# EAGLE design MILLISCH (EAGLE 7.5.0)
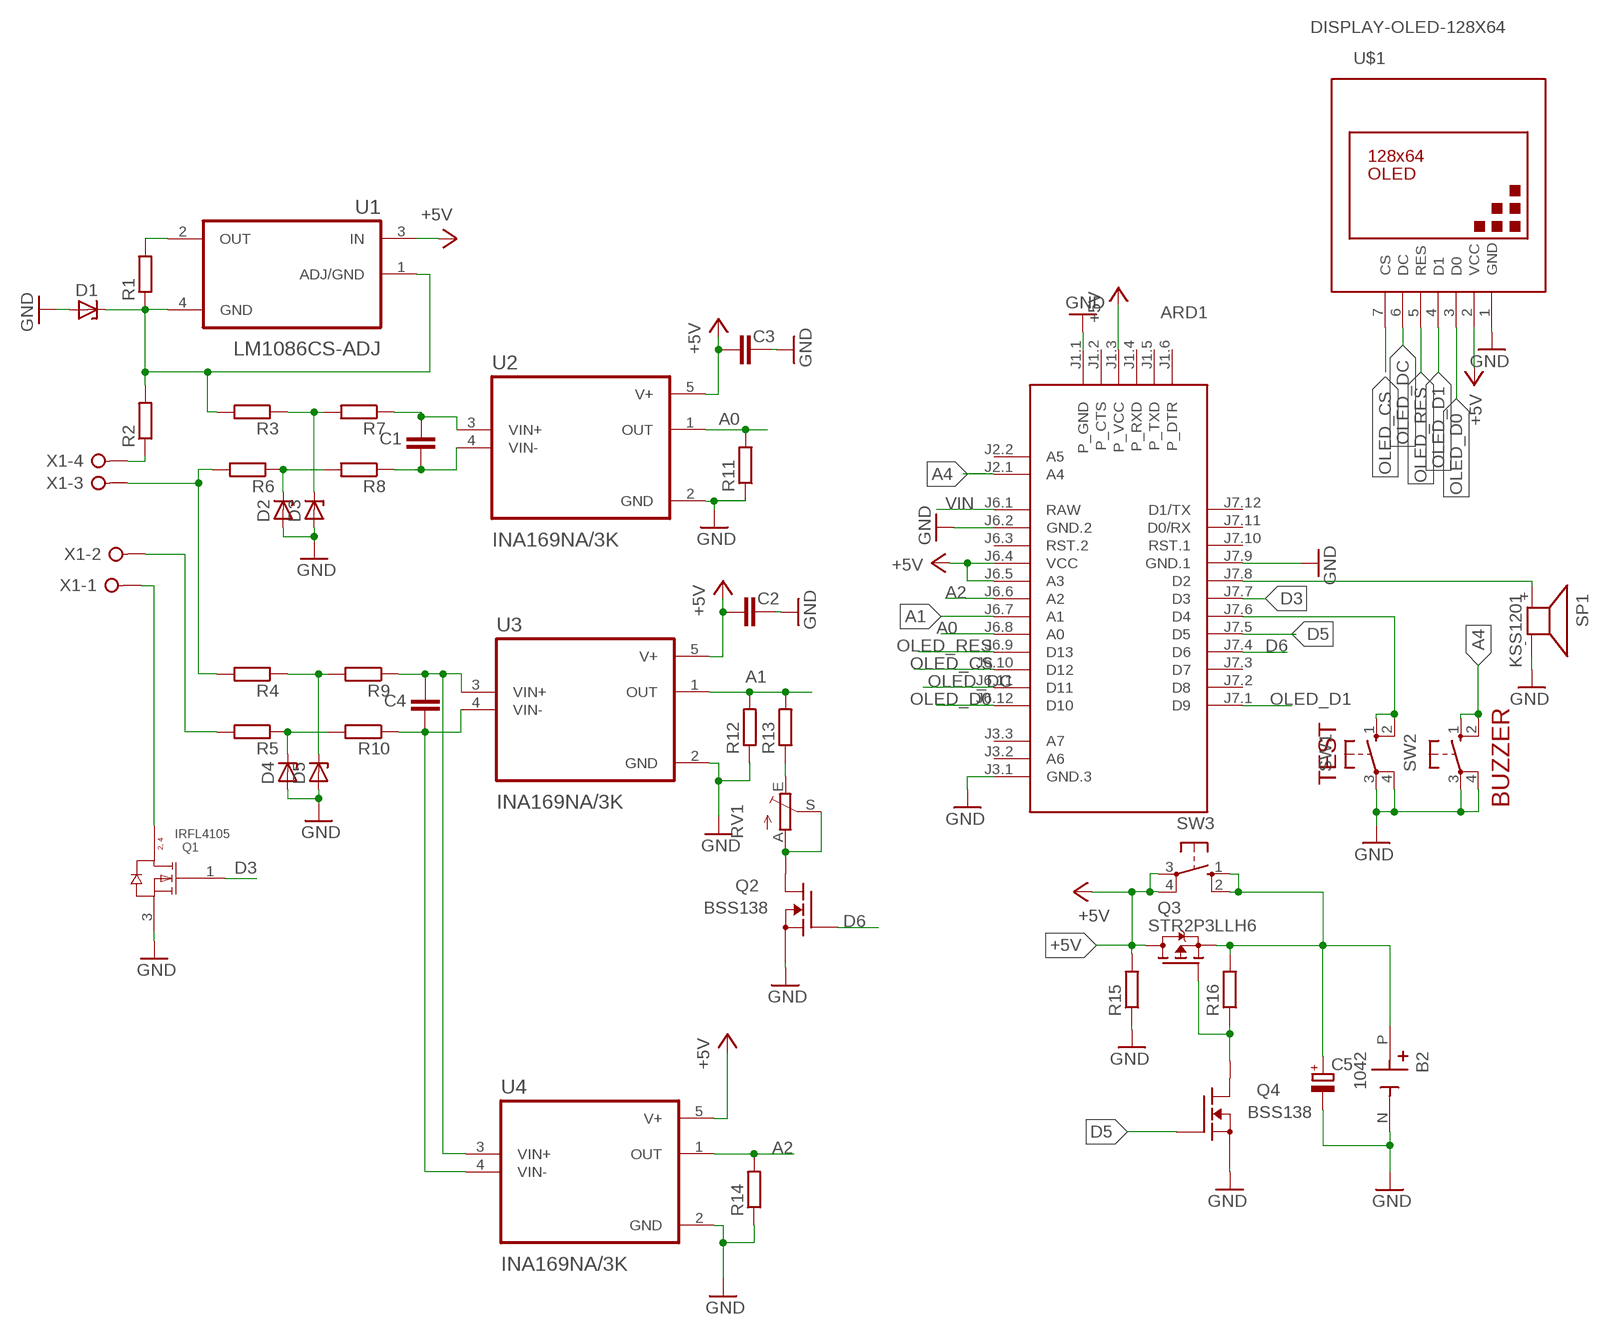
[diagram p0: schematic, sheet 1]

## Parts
ARD1  ARDUINO-PRO-MINI-3.3V  [ARDUINO-PRO-MINI]
B2  1042  [BAT_1042]
C1  C-EUC0805  [C0805]
C2  C-EUC0805  [C0805]
C3  C-EUC0805  [C0805]
C4  C-EUC0805  [C0805]
C5  CPOL-EUSMCD  [SMC_D]
D1  ZENER-DIODESMB  [SMB]
D2  ZENER-DIODESMB  [SMB]
D3  ZENER-DIODESMB  [SMB]
D4  ZENER-DIODESMB  [SMB]
D5  ZENER-DIODESMB  [SMB]
Q1  IRFL4105  NTF3055L108T1GNTF3055L108T1G_ONSC-SOT-223-4-318E-04_V  [ONSC-SOT-223-4-318E-04_V]
Q2  BSS138  [SOT23]
Q3  STR2P3LLH6  [SOT23]
Q4  BSS138  [SOT23]
R1  R-EU_R2512  [R2512]
R2  R-EU_R2512  [R2512]
R3  R-EU_R2512  [R2512]
R4  R-EU_R2512  [R2512]
R5  R-EU_R2512  [R2512]
R6  R-EU_R2512  [R2512]
R7  R-EU_R0805  [R0805]
R8  R-EU_R0805  [R0805]
R9  R-EU_R0805  [R0805]
R10  R-EU_R0805  [R0805]
R11  R-EU_R0805  [R0805]
R12  R-EU_R0805  [R0805]
R13  R-EU_R0805  [R0805]
R14  R-EU_R0805  [R0805]
R15  R-EU_R0805  [R0805]
R16  R-EU_R0805  [R0805]
RV1  TRIM_EU-B64W  [B64W]
SP1  KSS1201  [KSS1201]
SW1  10-XX  [B3F-10XX]
SW2  10-XX  [B3F-10XX]
SW3  10-XX  [B3F-10XX]
U1  LM1086CS-ADJ  [TO254P1524X483-4N]
U2  INA169NA/3K  [SOT95P280X145-5N]
U3  INA169NA/3K  [SOT95P280X145-5N]
U4  INA169NA/3K  [SOT95P280X145-5N]
U$1  DISPLAY-OLED-128X64  [DISPLAY-OLED-128X64]
X1  W237-04P  [W237-4P]

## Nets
+5V: ARD1.J1.3(P_VCC) ARD1.J6.4(VCC) ARD1.J6.5(A3) C2.1 C3.1 Q3.1(D) R15.2 SW3.3(P) SW3.4(P1) U1.3(IN) U2.5(V+) U3.5(V+) U4.5(V+) U$1.2(VCC)
A0: ARD1.J6.8(A0) R11.2 U2.1(OUT)
A1: ARD1.J6.7(A1) R12.2 R13.2 U3.1(OUT)
A2: ARD1.J6.6(A2) R14.2 U4.1(OUT)
A4: ARD1.J2.1(A4) SW2.1(S) SW2.2(S1)
D3: ARD1.J7.7(D3) Q1.1(G)
D5: ARD1.J7.5(D5) Q4.3(G)
D6: ARD1.J7.4(D6) Q2.3(G)
GND: ARD1.J1.1(P_GND) ARD1.J3.1(GND.3) ARD1.J6.2(GND.2) ARD1.J7.9(GND.1) B2.N(NEG) C2.2 C3.2 C5.- D1.A D2.A D3.A D4.A D5.A Q1.3(S) Q2.1(S) Q4.1(S) R11.1 R12.1 R14.1 R15.1 SP1.- SW1.3(P) SW1.4(P1) SW2.3(P) SW2.4(P1) U2.2(GND) U3.2(GND) U4.2(GND) U$1.1(GND)
N$1: C1.1 R7.1 U2.3(VIN+)
N$2: C1.2 R8.1 U2.4(VIN-)
N$3: R1.2 U1.2(OUT)
N$4: D1.C R1.1 R2.2 R3.2 U1.1(ADJ/GND) U1.4(GND)
N$5: R2.1 X1.4
N$6: R4.2 R6.2 X1.3
N$7: D3.C R3.1 R7.2
N$8: Q1.4(D) X1.1
N$9: D2.C R6.1 R8.2
N$10: C4.2 R10.1 U3.4(VIN-) U4.4(VIN-)
N$11: D5.C R4.1 R9.2
N$12: D4.C R5.1 R10.2
N$13: R5.2 X1.2
N$14: C4.1 R9.1 U3.3(VIN+) U4.3(VIN+)
N$15: Q2.2(D) RV1.A RV1.S
N$16: R13.1 RV1.E
N$17: ARD1.J7.8(D2) SP1.+
N$18: ARD1.J7.6(D4) SW1.1(S) SW1.2(S1)
N$19: Q3.2(G) Q4.2(D) R16.1
N$20: B2.P(POS) C5.+ Q3.3(S) R16.2 SW3.1(S) SW3.2(S1)
OLED_CS: ARD1.J6.10(D12) U$1.7(CS)
OLED_D0: ARD1.J6.12(D10) U$1.3(D0)
OLED_D1: ARD1.J7.1(D9) U$1.4(D1)
OLED_DC: ARD1.J6.11(D11) U$1.6(DC)
OLED_RES: ARD1.J6.9(D13) U$1.5(RES)
VIN: ARD1.J6.1(RAW)
Unconnected: ARD1.J1.2(P_CTS) ARD1.J1.4(P_RXD) ARD1.J1.5(P_TXD) ARD1.J1.6(P_DTR) ARD1.J2.2(A5) ARD1.J3.2(A6) ARD1.J3.3(A7) ARD1.J6.3(RST.2) ARD1.J7.2(D8) ARD1.J7.3(D7) ARD1.J7.10(RST.1) ARD1.J7.11(D0/RX) ARD1.J7.12(D1/TX) Q1.2(D)

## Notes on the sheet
- TEST
- BUZZER

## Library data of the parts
ARD1 = diy-modules:ARDUINO-PRO-MINI-*: Arduino Pro Mini and compatible devices More details available here: https://www.arduino.cc/en/Main/ArduinoBoardProMini Click here to find device on ebay.com
B2 = 18650-HOLDER:1042: Check availability; AVAILABILITY: In Stock; CHECK_PRICES: https://www.snapeda.com/parts/1042/Keystone/view-part/?ref=eda; DESCRIPTION: SMT Holder for 18650 Battery; MF: Keystone Electronics Corp.; MP: 1042; PACKAGE: NON STANDARD-5 Keystone; PRICE: None; SNAPEDA_LINK: https://www.snapeda.com/parts/1042/Keystone/view-part/?ref=snap
C1-C4 = rcl:C-EU: CAPACITOR, European symbol
C5 = rcl:CPOL-EU: POLARIZED CAPACITOR, European symbol
D1-D5 = diode:ZENER-DIODE: Z-Diode
Q1 = NTF3055L108T1G:NTF3055L108T1G: Power MOSFET, 3 A, 60 V, Logic Level, N-Channel, 4-Pin SOT-223, Pb-Free, Tape and Reel Check availability; AVAILABILITY: In Stock; CHECK_PRICES: https://www.snapeda.com/parts/NTF3055L108T1G/Onsemi/view-part/?ref=eda; DESCRIPTION: N-Channel 60 V 3A (Ta) 1.3W (Ta) Surface Mount SOT-223 (TO-261); MF: ON Semiconductor; MP: NTF3055L108T1G; PACKAGE: SOT-223-4 ON Semiconductor; PRICE: None; SNAPEDA_LINK: https://www.snapeda.com/parts/NTF3055L108T1G/Onsemi/view-part/?ref=snap
Q2 Q4 = transistor-fet:BSS138
Q3 = transistor-fet:STR2P3LLH6
R1-R16 = rcl:R-EU_: RESISTOR, European symbol
RV1 = pot:TRIM_EU-: POTENTIOMETER
SP1 = buzzer:KSS1201: SPEAKER; OC_FARNELL: unknown; OC_NEWARK: unknown
SW1-SW3 = switch-omron:10-XX: OMRON SWITCH; MPN: B3F-1000; OC_FARNELL: 176432; OC_NEWARK: 36M3542
U1 = LM1086CS-ADJ:LM1086CS-ADJ: Check availability; AVAILABILITY: In Stock; CHECK_PRICES: https://www.snapeda.com/parts/LM1086CS-ADJ/NOPB/Texas+Instruments/view-part/?ref=eda; DESCRIPTION: 1.5-A, 29-V, linear voltage regulator; MF: Texas Instruments; MP: LM1086CS-ADJ/NOPB; PACKAGE: TO263-3 Texas Instruments; PRICE: None; SNAPEDA_LINK: https://www.snapeda.com/parts/LM1086CS-ADJ/NOPB/Texas+Instruments/view-part/?ref=snap
U2-U4 = INA169NA_3K:INA169NA/3K: Check availability; AVAILABILITY: In Stock; CHECK_PRICES: https://www.snapeda.com/parts/INA169NA/3K/Texas+Instruments/view-part/?ref=eda; DESCRIPTION: 2.7 to 60V, 440kHz Variable gain current sense amplifier; MF: Texas Instruments; MP: INA169NA/3K; PACKAGE: SOT-23-5 Texas Instruments; PRICE: None; PURCHASE-URL: https://pricing.snapeda.com/search?q=INA169NA/3K&ref=eda; SNAPEDA_LINK: https://www.snapeda.com/parts/INA169NA/3K/Texas+Instruments/view-part/?ref=snap
U$1 = diy-modules:DISPLAY-OLED-128X64: 128x64 Dot Matrix OLED Module based on SSD1306 chip Variant with SPI interface More details available here: http://www.instructables.com/id/How-to-use-OLED-display-arduino-module/ SSD1306 datasheet: https://cdn-shop.adafruit.com/datasheets/SSD1306.pdf Click here to find device on ebay.com Note: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
X1 = con-wago-508:W237-04P: WAGO SREW CLAMP; OC_FARNELL: unknown; OC_NEWARK: unknown

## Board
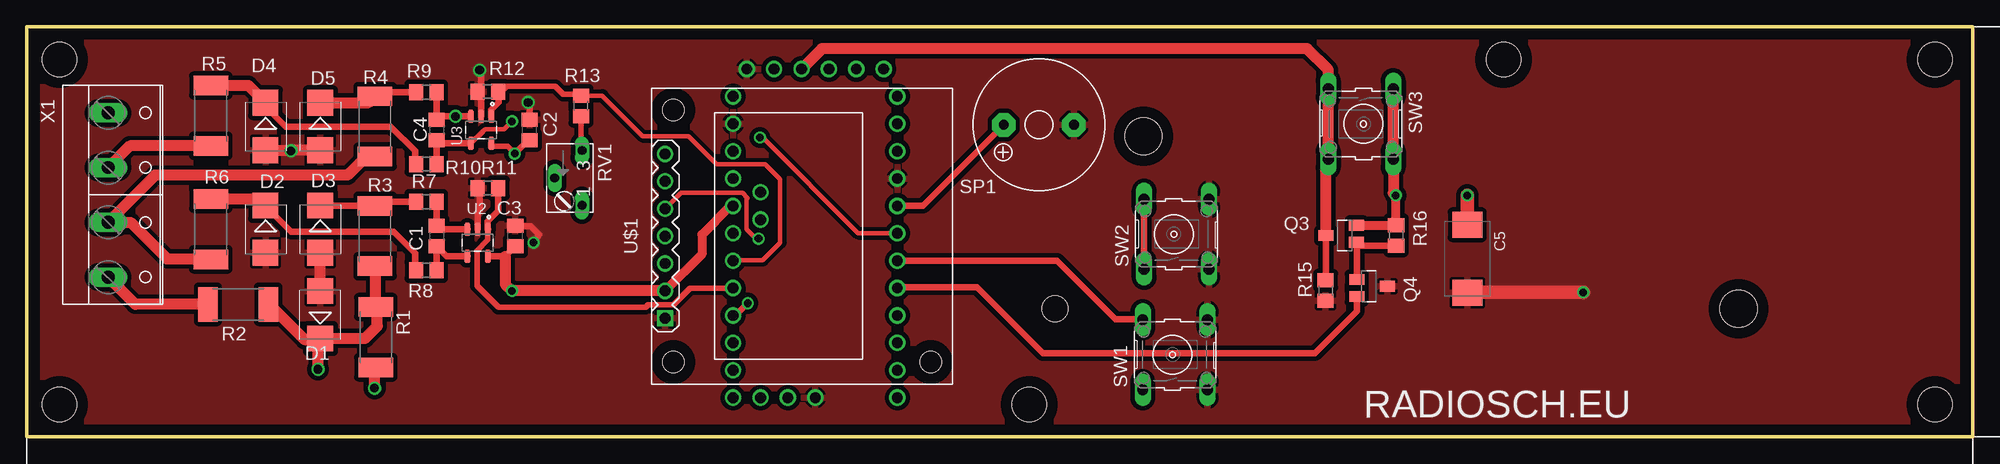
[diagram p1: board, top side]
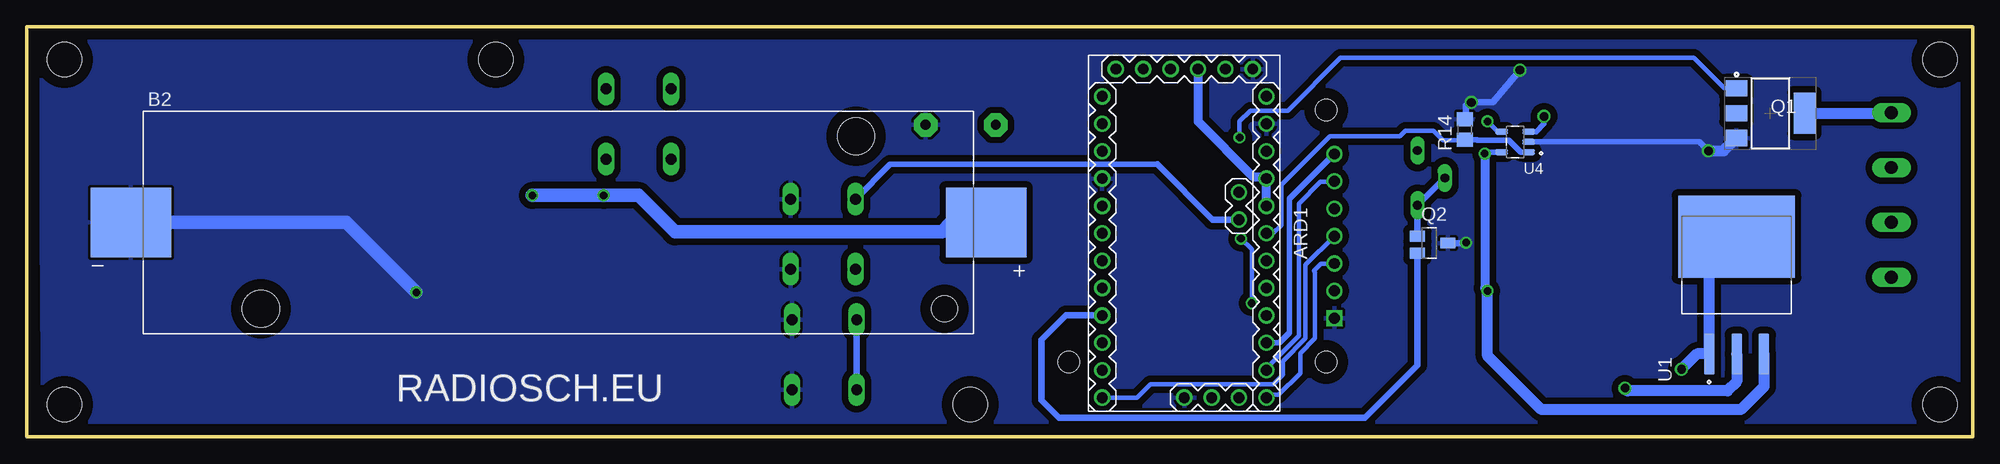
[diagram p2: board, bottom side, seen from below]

Size 180.5 x 38 mm. Coordinates in mm from the lower left corner, seen from the top.
Outline: 0,0 180.5,0 180.5,38 0,38 0,0
Copper layers (1*16): Top 0.035mm / dielectric 1.5mm / Bottom 0.035mm
Design rules "default": minimum track width 10mil, minimum drill 24mil, track to track 8mil, track to pad 8mil, pad to pad 8mil, via to via 8mil, smd to smd 8mil, copper to edge 40mil, drill to drill 8mil, minimum pad ring 10mil, minimum via ring 8mil, stop-mask expansion 4mil, vias tented up to drill 0mil, thermal gap 10mil
Holes 3.2 mm at 3,35 3,3 93,3 177,3 177,35 137,35

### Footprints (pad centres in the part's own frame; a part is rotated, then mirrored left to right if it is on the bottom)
ARDUINO-PRO-MINI = drill 1: J1.1 -15.24,6.35; J1.2 -15.24,3.81; J1.3 -15.24,1.27; J1.4 -15.24,-1.27; J1.5 -15.24,-3.81; J1.6 -15.24,-6.35; J2.1 -1.27,5.08; J2.2 -3.81,5.08; J3.1 15.24,0; J3.2 15.24,2.54; J3.3 15.24,5.08; J6.1 -12.7,7.62; J6.2 -10.16,7.62; J6.3 -7.62,7.62; J6.4 -5.08,7.62; J6.5 -2.54,7.62; J6.6 0,7.62; J6.7 2.54,7.62; J6.8 5.08,7.62; J6.9 7.62,7.62; J6.10 10.16,7.62; J6.11 12.7,7.62; J6.12 15.24,7.62; J7.1 15.24,-7.62; J7.2 12.7,-7.62; J7.3 10.16,-7.62; J7.4 7.62,-7.62; J7.5 5.08,-7.62; J7.6 2.54,-7.62; J7.7 0,-7.62; J7.8 -2.54,-7.62; J7.9 -5.08,-7.62; J7.10 -7.62,-7.62; J7.11 -10.16,-7.62; J7.12 -12.7,-7.62
BAT_1042 = smd 7.46 x 6.47: N -39.67,0; P 39.67,0 | hole 3.45: 27.6,8; -27.6,-8 | hole 2.39: 35.82,-8
C0805 = smd 1.3 x 1.5: 1 -0.95,0; 2 0.95,0
SMC_D = smd 2.4 x 2.8: + -3.15,0; - 3.15,0
SMB = smd 2.4 x 2.4: A 2.2,0; C -2.2,0
ONSC-SOT-223-4-318E-04_V = smd 2 x 1.5: 1 -3.15,2.3; 2 -3.15,0; 3 -3.15,-2.3 | smd 2 x 3.8: 4 3.15,0
SOT23 = smd 1 x 1.4: 1 0,1.735; 2 -0.632,-1.1; 3 0.95,-1.1
R2512 = smd 1.8 x 3.2: 1 -2.8,0; 2 2.8,0
R0805 = smd 1.3 x 1.5: 1 -0.95,0; 2 0.95,0
B64W = drill 0.813 long: A 2.54,0; E -2.54,0; S 0,-2.54
KSS1201 = drill 0.914 pad 2.159 octagon: + 3.251,0; - -3.251,0
B3F-10XX = drill 1.016 long: 1 -3.251,2.761; 2 3.251,2.761; 3 -3.251,-3.261; 4 3.251,-3.261
TO254P1524X483-4N = smd 3.79 x 0.99: 1 -6.4,2.54; 2 -6.4,0; 3 -6.4,-2.54 | smd 7.62 x 10.84: 4 4.48,0
SOT95P280X145-5N = smd 1.21 x 0.59: 1 -1.255,0.95; 2 -1.255,0; 3 -1.255,-0.95; 4 1.255,-0.95; 5 1.255,0.95
DISPLAY-OLED-128X64 = drill 1 square: 1 -7.62,12.7 | drill 1: 2 -5.08,12.7; 3 -2.54,12.7; 4 0,12.7; 5 2.54,12.7; 6 5.08,12.7; 7 7.62,12.7 | hole 2: -11.684,11.938; 11.684,11.938; -11.684,-11.938
W237-4P = drill 1.194 long: 1 -7.62,-0.635; 2 -2.54,-0.635; 3 2.54,-0.635; 4 7.62,-0.635

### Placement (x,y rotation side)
ARD1  73.13,18.86 270 bottom
B2  131.19,19.87 0 bottom
C1  38.01,18.61 270 top
C2  46.62,28.45 90 top
C3  45.31,18.61 90 top
C4  38.01,28.45 270 top
C5  133.62,16.5 270 top
D1  27.21,11.31 90 top
D2  22.13,19.25 270 top
D3  27.21,19.25 270 top
D4  22.13,28.77 270 top
D5  27.21,28.77 270 top
Q1  18.75,30 0 bottom
Q2  50.41,17.95 270 bottom
Q3  122.25,18.66 90 top
Q4  124.48,13.95 270 top
R1  32.37,9.22 270 top
R2  19.59,12.26 0 top
R3  32.29,18.61 270 top
R4  32.29,28.77 270 top
R5  17.05,29.77 270 top
R6  17.05,19.25 270 top
R7  37.05,21.79 180 top
R8  37.05,15.44 180 top
R9  37.05,31.95 180 top
R10  37.05,25.28 180 top
R11  42.77,23.05 0 top
R12  42.75,32 0 top
R13  51.4,30.68 90 top
R14  47.11,28.47 270 bottom
R15  120.47,13.54 90 top
R16  127.02,18.67 90 top
RV1  51.5,24 270 top
SP1  93.88,28.91 180 top
SW1  106.28,7.61 90 top
SW2  106.4,18.79 90 top
SW3  124,29 270 top
U1  21.89,14.07 90 bottom
U2  41.81,17.98 270 top
U3  42.13,28.45 270 top
U4  42.44,27.34 180 bottom
U$1  71.91,18.6 90 top
X1  8.16,22.42 270 top

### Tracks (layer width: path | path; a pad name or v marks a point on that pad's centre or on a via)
+5V  (via drill 0.7)
  Top 0.5: 43.08,26.92 44.58,26.92 v45.25,26.25 46.5,27.5 C2.1
  Top 0.61: U2.5 44.37,16.72 C3.1 | U3.5 43.08,26.92 | Q3.1 120.52,14.54 R15.2
  Top 0.813: ARD1.J6.5 65.28,21.4 62.62,18.75 62.62,16.94 U$1.2
  Top 1.016: 44.37,16.72 44.37,14.15 v45,13.52 U$1.2 | ARD1.J1.3 73.76,36 118.75,36 120.74,34.01 SW3.3 SW3.4 120.52,25.53 Q3.1
  Bottom 0.5: U4.5 45.11,26.39 v45.25,26.25
  Bottom 0.813: v45.25,26.25 45.25,13.77 v45,13.52 | ARD1.J6.5 ARD1.J6.4 65.69,24.12 66.75,24.12 71.86,29.23 ARD1.J1.3
  Bottom 1.016: U1.3 19.35,4.65 21.5,2.5 40,2.5 45,7.5 v45,13.52
A0
  Top 0.5: ARD1.J6.8 61.53,13.78 60,12.25 57.62,12.25 57.38,12 43.75,12 41.75,14 41.75,17.25 42.75,18.25 42.75,19.21 U2.1
  Top 0.61: R11.2 43.72,20.97 42.75,20 42.75,19.25 U2.1
A1
  Top 0.406: R13.2 53.37,31.63 57.12,27.88 61.38,27.88 64,25.25 68.5,25.25 69.88,23.88 69.88,18 68.25,16.38 65.56,16.38 ARD1.J6.7
  Top 0.5: 43.75,31.95 43.95,31.95 44.5,32.5 49,32.5 49.75,31.75 51.28,31.75 R13.2
  Top 0.61: U3.1 43.08,30.33 43.75,31 43.75,31.95 R12.2
A2
  Bottom 0.406: ARD1.J6.6 64.89,18.86 64.12,19.62 64.12,23.38 59.62,27.88 53.12,27.88 52.62,28.38 50,28.38 49.12,27.5 47.13,27.5 R14.2
  Bottom 0.5: R14.2 45.98,27.52 45.96,27.5 43,27.5 41.89,26.39 U4.1
A4
  Top 0.61: SW2.2 SW2.1
  Bottom 0.5: 75.62,25.25 100.43,25.25 SW2.2
  Bottom 0.61: ARD1.J2.1 70.5,20.13 75.62,25.25
D3  (via drill 0.7)
  Top 0.406: v68,27.75 68.25,27.75 77.12,18.88 80.73,18.88 ARD1.J7.7
  Bottom 0.406: Q1.1 23.05,32.3 25.88,35.12 58.62,35.12 63.5,30.25 67,30.25 68,29.25 v68,27.75
D5
  Top 0.61: Q4.3 123.38,11.63 119.5,7.75 94.25,7.75 88.12,13.88 80.84,13.88 ARD1.J7.5
D6
  Bottom 0.61: Q2.3 51.51,6.62 56.38,1.75 84.75,1.75 86.38,3.38 86.38,9 84.12,11.25 ARD1.J7.4
GND  (via drill 0.7, 0.8)
  Top 0.5: U3.2 42.13,31.67 R12.1
  Top 0.61: U3.2 42.13,33.37 v42,34 | C2.2 46.62,30.88 v46.5,31 | U2.2 41.81,20.82 42,21 42,22.87 R11.1 | v47,18 47.5,18.75 46.75,19.5 45.37,19.5 C3.2
  Top 1.016: D1.A D3.A | D4.A 24.43,26.57 v24.5,26.5 24.57,26.57 D5.A
  Top 1.27: v144.38,13.38 133.65,13.38 C5.-
  Bottom 0.5: U4.2 25.34,27.34 v24.5,26.5
  Bottom 0.61: v42,34 44.5,31 v46.5,31 46.75,31 47,30.75 47,29.53 R14.1 | Q2.1 47.55,17.95 v47,18
  Bottom 1.016: v24.5,26.5 23.1,26.5 Q1.3
  Bottom 1.27: B2.N 150.87,19.87 v144.38,13.38
  pour Top (isolate 0.406): 1,37 179.75,37 179.25,0.5 1.5,0.5
  pour Bottom (isolate 0.61): 1.25,37.5 179.25,37.5 179,0.5 1,0.5
N$1
  Top 0.61: R7.1 C1.1 38.34,19.23 U2.3
N$2
  Top 0.61: R8.1 C1.2 38.95,16.72 U2.4
N$3  (via drill 0.8)
  Top 1.016: v32.25,4.5 32.25,6.3 R1.2
  Bottom 1.016: U1.2 21.89,5.11 22.75,4.25 32,4.25 v32.25,4.5
N$4  (via drill 0.8)
  Top 1.016: R3.2 32.37,15.73 R1.1 32.5,11.89 32.5,10.25 31.36,9.11 D1.C | R2.2 22.49,12.26 25.75,9 27.1,9 D1.C | v27,6.25 27,8.9 D1.C
  Bottom 1.016: U1.4 24.43,16.01 U1.1 25.58,7.67 v27,6.25
N$5
  Top 1.016: R2.1 10.06,12.26 X1.4
N$6
  Top 1.016: R6.2 17,16.5 13,16.5 9.62,19.88 X1.3 11.89,24.25 29.75,24.25 31.47,25.97 R4.2
N$7
  Top 0.61: R7.2 32.66,21.79 R3.1 27.25,21.41 D3.C
N$8
  Bottom 1.016: Q1.4 7.57,30 X1.1
N$9
  Top 0.61: D2.C 22.13,21.37 24.5,19 34,19 36,17 36,15.54 R8.2
  Top 1.016: R6.1 21.53,22.05 D2.C
N$10  (via drill 0.7)
  Top 0.406: 42.23,28.25 42.25,28.25 42.5,28.5 44.25,28.5 v45,29.25
  Top 0.5: 42.23,28.25 U3.4
  Top 0.61: R10.1 C4.2 38.31,27.2 U3.4
  Bottom 0.406: U4.4 44.04,28.29 v45,29.25
N$11
  Top 0.61: R9.2 32.66,31.95 R4.1
  Top 1.016: D5.C 31.69,30.97 R4.1
N$12
  Top 0.61: D4.C 22.13,30.62 24,28.75 33.75,28.75 36,26.5 36,25.38 R10.2
  Top 1.016: R5.1 20.53,32.57 D4.C
N$13
  Top 1.016: R5.2 9.54,26.97 X1.2
N$14  (via drill 0.8)
  Top 0.61: R9.1 C4.1 38.31,29.71 v39.75,29.71 U3.3
  Bottom 0.5: U4.3 40.46,28.29 39.75,29 v39.75,29.71
N$15
  Bottom 0.61: Q2.2 RV1.A RV1.S
N$16
  Top 0.5: 51.52,26.56 RV1.E 51.4,26.64 R13.1
N$17
  Top 0.61: ARD1.J7.8 83.11,21.4 SP1.+
N$18
  Top 0.61: ARD1.J7.6 95.56,16.32 101,10.88 103.5,10.88 SW1.2
  Bottom 0.61: SW1.2 SW1.1
N$19
  Top 0.61: Q4.2 123.38,18.01 Q3.2 123.67,17.72 R16.1
N$20  (via drill 0.7)
  Top 0.813: v127,22.38 127.02,22.36 R16.2 Q3.3
  Top 1.016: v127,22.38 126.76,22.61 SW3.2 SW3.1
  Top 1.27: v133.62,22.38 C5.+
  Bottom 1.27: B2.P 94.75,19.87 95.62,19 120.38,19 123.75,22.38 v127,22.38 v133.62,22.38
OLED_CS
  Bottom 0.5: ARD1.J6.10 64.3,8.7 63.38,9.62 63.38,22.05 U$1.7
OLED_D0
  Bottom 0.406: U$1.3 60.44,16.06 61.12,15.38 61,15.25 61,9.12 62.38,7.75 62.38,5.88 64.38,3.88 65.25,3.88 ARD1.J6.12
OLED_D1
  Bottom 0.406: ARD1.J7.1 77.5,3.62 76.25,4.88 64.88,4.88 64,5.75 64,7 61.88,9.12 61.88,15.94 U$1.4
OLED_DC
  Bottom 0.406: ARD1.J6.11 65.51,6.37 62.5,9.38 62.5,21.62 60.5,23.62 59.27,23.62 U$1.6
OLED_RES  (via drill 0.7)
  Top 0.406: U$1.5 60.7,22.62 66.38,22.62 66.88,22.12 66.75,22 66.75,19.25 67.62,18.38 v67.88,18.38
  Top 0.5: ARD1.J6.9 65.74,11.24 v66.88,12.38
  Bottom 0.406: v66.88,12.38 66.88,17.38 v67.88,18.38

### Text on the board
tPlace: RADIOSCH.EU
bPlace: RADIOSCH.EU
